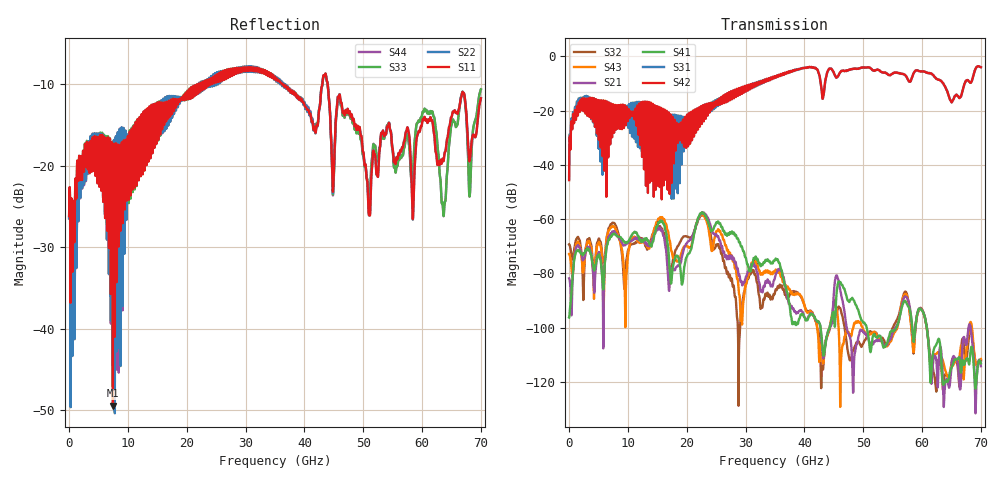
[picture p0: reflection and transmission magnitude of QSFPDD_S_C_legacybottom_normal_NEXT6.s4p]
! AWR Design Environment (8415) Thu Dec 20 14:56:50 2018
! Document = 'CHANNEL TEST'
! nPorts: 4, nXvals: 7001
# HZ S DB R 50
!Freq DBS11 AngS11 DBS12 AngS12 DBS13 AngS13 DBS14 AngS14
!	DBS21 AngS21 DBS22 AngS22 DBS23 AngS23 DBS24 AngS24
!	DBS31 AngS31 DBS32 AngS32 DBS33 AngS33 DBS34 AngS34
!	DBS41 AngS41 DBS42 AngS42 DBS43 AngS43 DBS44 AngS44
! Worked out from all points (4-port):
!   7000 points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, 10 MHz to 70 GHz, reference 50 ohm
!   strongest paths, dB at 10 MHz, 17.51 GHz, 35.01 GHz, 52.51 GHz, 70 GHz:
!     S42: -45.6, -25.5, -7.4, -5.0, -4.0
!     S31: -45.3, -28.7, -7.5, -5.0, -4.0
!     S41: -96.3, -79.8, -75.0, -103.3, -113.2
!     S21: -81.8, -78.1, -81.4, -104.7, -114.2
!     S43: -72.9, -72.5, -79.3, -103.5, -111.5
!     S32: -69.3, -76.8, -87.0, -103.4, -112.3
!   lowest |S11| = -49.4 dB at 7.45 GHz (marker M1), VSWR 1.01, Z = 50.3 + j0.0931 ohm
!   |S11| at or under -10 dB: start of sweep to 22.1 GHz; 36.25 GHz to 43.06 GHz (6.813 GHz wide, 17.2 % of centre); 43.96 GHz to end of sweep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
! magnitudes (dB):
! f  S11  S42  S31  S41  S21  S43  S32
! 10 MHz  -26.2  -45.6  -45.3  -96.3  -81.8  -72.9  -69.3
! 1.64 GHz  -19.9  -17.1  -15.5  -71.9  -70.2  -69.0  -67.2
! 7.45 GHz  -49.4  -18.1  -18.5  -65.6  -64.6  -62.7  -61.3
! 9.42 GHz  -22.1  -19.1  -22.3  -68.3  -69.5  -82.8  -85.5
! 22.65 GHz  -10.7  -20.1  -21.9  -57.5  -57.6  -58.2  -58.3
! 27.13 GHz  -8.3  -14.2  -14.0  -65.7  -74.7  -72.6  -81.4
! 70 GHz  -11.8  -4.0  -4.0  -113.2  -114.2  -111.5  -112.3
